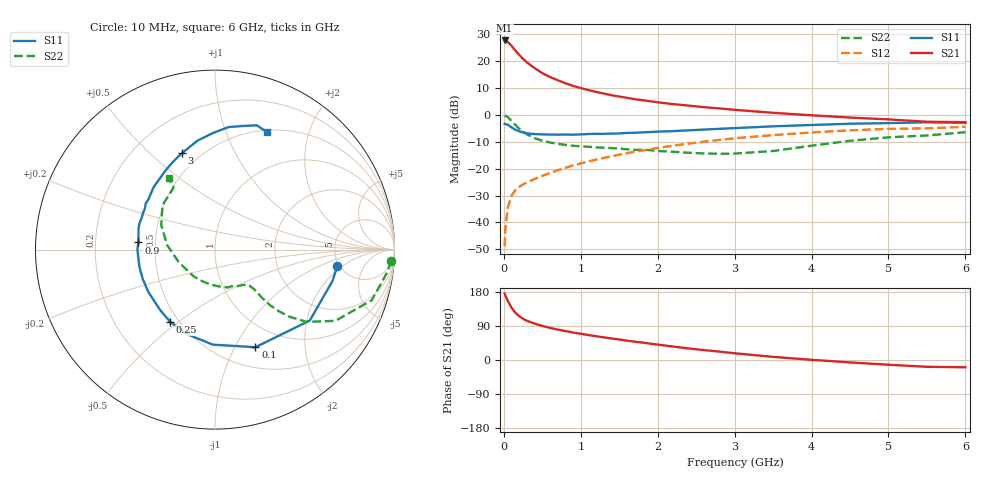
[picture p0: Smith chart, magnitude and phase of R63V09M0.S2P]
! SIEMENS Small Signal Semiconductors
! BFR193
! Si NPN RF Bipolar Junction Transistor in SOT23
! VCE = 3 V  IC = 9 mA
! Common Emitter S-Parameters:  May  1996
# GHz  S  MA  R  50
!  f  S11  S21  S12  S22
! GHz  MAG  ANG  MAG  ANG  MAG  ANG  MAG  ANG
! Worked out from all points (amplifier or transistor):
!   36 points, 10 MHz to 6 GHz, reference 50 ohm
!   highest |S21| = 27.8 dB at 10 MHz (marker M1)
!   |S21| within 3 dB of that: start of sweep to 129 MHz
!   unconditionally stable (mu >= 1): 758.8 MHz to 1.931 GHz
!   at 250 MHz: K = 0.61, MSG = 23.4 dB, |S12| = -25.9 dB
!   at 1.4 GHz: K = 1.04, MAG = 10.1 dB, |S12| = -15.4 dB
!   at 6 GHz: K = 0.95, MSG = 0.9 dB, |S12| = -4.4 dB
!   S11 on the Smith chart (normalised r, x): 10 MHz: 4.78, -1.69; 100 MHz: 0.73, -1.21; 250 MHz: 0.45, -0.47; 900 MHz: 0.40, +0.04; 3 GHz: 0.40, +0.64; 6 GHz: 0.53, +1.41
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0.01  0.6875 -7.8  24.42 175.2  0.0036 87.1  0.9842 -3.7
0.02  0.6775 -15.0  24.42 170.1  0.0077 82.1  0.9677 -7.5
0.05  0.6595 -36.8  23.05 156.5  0.0184 74.0  0.9176 -17.9
0.1  0.5887 -67.5  19.38 138.3  0.0314 63.4  0.7796 -30.6
0.15  0.5297 -91.3  15.92 124.5  0.0398 57.0  0.6499 -38.3
0.2  0.4964 -108.0  13.15 115.7  0.0458 55.1  0.5547 -42.2
0.25  0.4736 -121.9  11.08 108.7  0.0509 54.1  0.4863 -44.2
0.3  0.4546 -132.2  9.554 103.5  0.0553 54.4  0.4351 -45.3
0.4  0.4402 -147.5  7.443 96.1  0.0642 56.4  0.3695 -45.7
0.5  0.4345 -158.2  6.029 90.0  0.0734 57.7  0.331 -45.4
0.6  0.432 -167.1  5.101 84.7  0.0831 59.2  0.307 -45.4
0.7  0.4298 -174.8  4.438 80.2  0.0933 60.3  0.2906 -45.9
0.9  0.429 174.7  3.487 72.6  0.1151 61.9  0.2667 -47.4
1.1  0.4421 164.6  2.907 65.9  0.136 62.0  0.2555 -50.6
1.4  0.45 152.6  2.333 56.7  0.17 61.2  0.2417 -57.0
1.6  0.4637 146.2  2.085 51.0  0.194 60.0  0.2296 -62.7
2.2  0.5005 128.2  1.592 35.5  0.2678 54.5  0.2062 -84.1
3  0.5684 108.8  1.248 17.7  0.3675 44.0  0.1908 -128.4
3.5  0.615 99.1  1.097 8.3  0.4219 36.3  0.2132 -160.3
4.5  0.6868 83.7  0.894 -6.4  0.518 21.2  0.33 155.3
5.5  0.7308 71.4  0.747 -17.9  0.5638 5.5  0.4151 123.8
6  0.7152 65.9  0.736 -19.2  0.6017 0.9  0.4768 122.7
